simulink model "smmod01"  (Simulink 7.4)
settings: Solver=ode45  StartTime=0.0  StopTime=3  MaxStep=5e-4  RelTol=1e-4  AbsTol=1e-4
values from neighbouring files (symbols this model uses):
  Bm = 0.10    (= 0.1)    [IMabc2.m]    (also in imabcparam.m = 0.01; IMabcrun0.m = 0.01; IMabcrun1.m = 0.001; IMcur0.m = 1e-06)
  H = 0.60    (= 0.6)    [IMabc2.m]    (also in IMcur0.m = 0.3; imdef0vec.m = 0.3; imdef1vec.m = 0.3; imdef2vec.m = 0.3)
  n0 = 0.98    [imdef0vec.m]    (also in imdef1vec.m = 0.978; imdef2vec.m; imdefrotflux.m; imdefSIvec1.m = 0.95)
  Ra = .95    (= 0.95)    [altwdgs.m]    (also in Ccurverun.m = 0.018)
  Te0 = 0.75/wo*p*(Is*conj(Is)*Req)    [imdefSIvec1.m]
  V = [Vas 0 0].'    [Actac.m]    (also in acttrcalc1.m = str2num(get(h,'string')); im3d.m = eval(get(hVs,'String')); IMabc2.m = [vas vbs vcs 0 0 0]'; IMabcf0.m = [vas vbs vcs 0 0 0]')
  wo = 2*pi*freq0    [calc0.m]    (also in IMabc2.m = 376.991118431; imabcparam.m = 376.991118431; IMabcrun0.m = 376.991118431; IMabcrun1.m = 376.991118431)
undefined symbols (not defined in the file or in its folder): delta0, fa0, fk0, Lal, Lfl, Lkdl, Lkql, Lmd, Lmq, ph, phif0, Rf, Rkd, Rkq, vf0

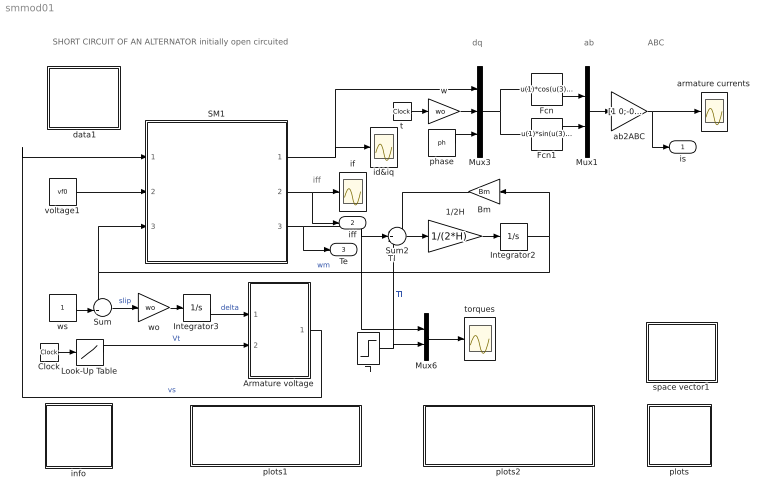
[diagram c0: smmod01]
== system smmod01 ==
  note: Tl
  note: SHORT CIRCUIT OF AN ALTERNATOR initially open circuited
  note: iff
  note: dq
  note: ab
  note: ABC
  " data1" : Subsystem
  1/2H : Gain  Gain=1/(2*H)  ParameterDataType=sfix(16)  ParameterScaling=2^0  OutDataType=sfix(16)  OutScaling=2^0
  Armature voltage : Subsystem
  Bm : Gain  Gain=Bm  ParameterDataType=sfix(16)  ParameterScaling=2^0  OutDataType=sfix(16)  OutScaling=2^0
  Clock : Clock
  Fcn : Fcn  Expr=u(1)*cos(u(3)+u(4))-u(2)*sin(u(3)+u(4))
  Fcn1 : Fcn  Expr=u(1)*sin(u(3)+u(4))+u(2)*cos(u(3)+u(4))
  Integrator2 : Integrator  InitialCondition=n0
  Integrator3 : Integrator  InitialCondition=delta0
  Look-Up Table : Lookup  InputValues=[0 0.2 0.2 5]  Table=[V V 0 0]  OutDataType=sfix(16)  OutScaling=2^0
  Mux1 : Mux  Inputs=2
  Mux3 : Mux  Inputs=3
  Mux6 : Mux  Inputs=2
  SM1 : Subsystem
  Sum : Sum  Inputs=-+|  OutDataType=sfix(16)  OutScaling=2^0
  Sum2 : Sum  Inputs=-+-  OutDataType=sfix(16)  OutScaling=2^0
  Tl : Step  Time=0  After=Te0  SampleTime=0
  ab2ABC : Gain  Gain=[1 0;-0.5 sqrt(3)/2;-0.5 -sqrt(3)/2]  Multiplication=Matrix(K*u)  ParameterDataType=sfix(16)  ParameterScaling=2^0  OutDataType=sfix(16)  OutScaling=2^0
  armature currents : Scope
  id&iq : Scope
  if : Scope
  info : Subsystem
  phase : Constant  Value=ph  OutDataType=sfix(16)  OutScaling=2^0
  plots : Subsystem
  plots1 : Subsystem
  plots2 : Subsystem
  space vector1 : Subsystem
  t : Clock
  torques : Scope
  voltage1 : Constant  Value=vf0  OutDataType=sfix(16)  OutScaling=2^0
  w : Gain  Gain=wo  ParameterDataType=sfix(16)  ParameterScaling=2^0  OutDataType=sfix(16)  OutScaling=2^0
  wo : Gain  Gain=wo  ParameterDataType=sfix(16)  ParameterScaling=2^0  OutDataType=sfix(16)  OutScaling=2^0
  ws : Constant  OutDataType=sfix(16)  OutScaling=2^0
  is : Outport
  iff : Outport  Port=2
  Te : Outport  Port=3
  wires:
  voltage1/1 -> SM1/2(vf)
  1/2H/1 -> Integrator2/1
  Sum2/1 -> 1/2H/1
  Bm/1 -> Sum2/1
  Mux6/1 -> torques/1
  ws/1 -> Sum/2
  Sum/1 -> wo/1  "slip"
  Armature voltage/1(vs) -> SM1/1(vs)  "vs"
  wo/1 -> Integrator3/1
  Integrator3/1 -> Armature voltage/1(delta)  "delta"
  Clock/1 -> Look-Up Table/1
  Look-Up Table/1 -> Armature voltage/2(Vt)  "Vt"
  Integrator2/1 -> Bm/1, Sum/1, SM1/3(wm)  "wm"
  w/1 -> Mux3/2
  phase/1 -> Mux3/3
  t/1 -> w/1
  SM1/2(if) -> if/1, iff/1
  SM1/3(Te) -> Sum2/2, Mux6/1, Te/1
  SM1/1(ia) -> id&iq/1, Mux3/1
  Tl/1 -> Mux6/2, Sum2/3  "Tl"
  Mux3/1 -> Fcn/1, Fcn1/1
  Fcn1/1 -> Mux1/2
  Fcn/1 -> Mux1/1
  Mux1/1 -> ab2ABC/1
  ab2ABC/1 -> armature currents/1, is/1

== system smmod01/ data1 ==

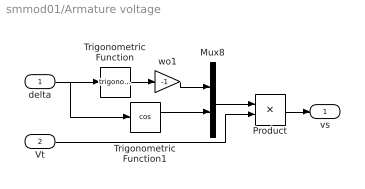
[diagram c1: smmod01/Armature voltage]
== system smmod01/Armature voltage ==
  delta : Inport  OutDataType=sfix(16)  OutScaling=2^0
  Vt : Inport  Port=2  OutDataType=sfix(16)  OutScaling=2^0
  Mux8 : Mux  Inputs=2
  Product : Product  OutDataType=sfix(16)  OutScaling=2^0
  Trigonometric Function : Trigonometry
  Trigonometric Function1 : Trigonometry  Operator=cos
  wo1 : Gain  Gain=-1  ParameterDataType=sfix(16)  ParameterScaling=2^0  OutDataType=sfix(16)  OutScaling=2^0
  vs : Outport
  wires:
  delta/1 -> Trigonometric Function/1, Trigonometric Function1/1
  Trigonometric Function/1 -> wo1/1
  Mux8/1 -> Product/1
  wo1/1 -> Mux8/1
  Trigonometric Function1/1 -> Mux8/2
  Product/1 -> vs/1
  Vt/1 -> Product/2

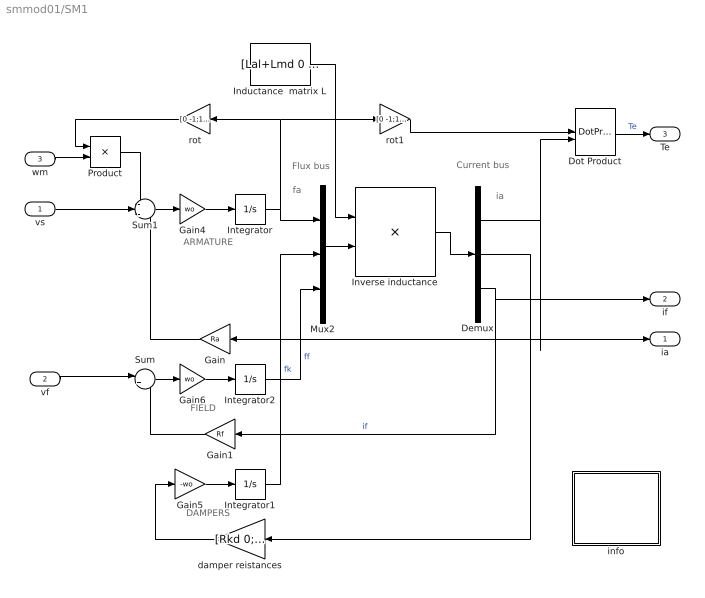
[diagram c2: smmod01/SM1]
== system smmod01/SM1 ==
  note: DAMPERS
  note: ARMATURE
  note: fa
  note: ia
  note: FIELD
  note: Flux bus
  note: Current bus
  vs : Inport  OutDataType=sfix(16)  OutScaling=2^0
  vf : Inport  Port=2  OutDataType=sfix(16)  OutScaling=2^0
  wm : Inport  Port=3  OutDataType=sfix(16)  OutScaling=2^0
  Demux : Demux  Outputs=3
  Dot Product : DotProduct  OutDataType=fixdt(1, 16)  OutScaling=2^-10
  Gain : Gain  Gain=Ra  ParameterDataType=sfix(16)  ParameterScaling=2^0  OutDataType=sfix(16)  OutScaling=2^0
  Gain1 : Gain  Gain=Rf  ParameterDataType=sfix(16)  ParameterScaling=2^0  OutDataType=sfix(16)  OutScaling=2^0
  Gain4 : Gain  Gain=wo  ParameterDataType=sfix(16)  ParameterScaling=2^0  OutDataType=sfix(16)  OutScaling=2^0
  Gain5 : Gain  Gain=-wo  ParameterDataType=sfix(16)  ParameterScaling=2^0  OutDataType=sfix(16)  OutScaling=2^0
  Gain6 : Gain  Gain=wo  ParameterDataType=sfix(16)  ParameterScaling=2^0  OutDataType=sfix(16)  OutScaling=2^0
  Inductance  matrix L : Constant  Value=[Lal+Lmd 0 Lmd 0 Lmd;0 Lal+Lmq 0 Lmq 0;Lmd 0 Lmd+Lkdl 0 Lmd;0 Lmq 0 Lmq+Lkql 0;Lmd 0 Lmd 0 Lmd+Lfl]  VectorParams1D=off  OutDataType=fixdt(1, 16)  OutScaling=2^0
  Integrator : Integrator  InitialCondition=fa0
  Integrator1 : Integrator  InitialCondition=fk0
  Integrator2 : Integrator  InitialCondition=phif0
  Inverse inductance : Product  Inputs=/*  Multiplication=Matrix(*)  OutDataType=sfix(16)  OutScaling=2^0
  Mux2 : Mux  Inputs=3
  Product : Product  OutDataType=sfix(16)  OutScaling=2^0
  Sum : Sum  Inputs=|+-  OutDataType=sfix(16)  OutScaling=2^0
  Sum1 : Sum  Inputs=-+-  OutDataType=sfix(16)  OutScaling=2^0
  damper reistances : Gain  Gain=[Rkd 0;0 Rkq]  Multiplication=Matrix(K*u)  ParameterDataType=sfix(16)  ParameterScaling=2^0  OutDataType=sfix(16)  OutScaling=2^0
  info : Subsystem
  rot : Gain  Gain=[0 -1;1 0]  Multiplication=Matrix(K*u)  ParameterDataType=sfix(16)  ParameterScaling=2^0  OutDataType=sfix(16)  OutScaling=2^0
  rot1 : Gain  Gain=[0 -1;1 0]  Multiplication=Matrix(K*u)  ParameterDataType=sfix(16)  ParameterScaling=2^0  OutDataType=sfix(16)  OutScaling=2^0
  ia : Outport
  if : Outport  Port=2
  Te : Outport  Port=3
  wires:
  Product/1 -> Sum1/1
  rot/1 -> Product/1
  wm/1 -> Product/2
  Gain5/1 -> Integrator1/1
  damper reistances/1 -> Gain5/1
  Integrator/1 -> Mux2/1, rot/1, rot1/1
  Sum1/1 -> Gain4/1
  Gain4/1 -> Integrator/1
  vs/1 -> Sum1/2
  Gain/1 -> Sum1/3
  Gain6/1 -> Integrator2/1
  Sum/1 -> Gain6/1
  vf/1 -> Sum/1
  Gain1/1 -> Sum/2
  rot1/1 -> Dot Product/1
  Demux/1 -> Gain/1, ia/1, Dot Product/2
  Dot Product/1 -> Te/1  "Te"
  Integrator1/1 -> Mux2/2  "fk"
  Integrator2/1 -> Mux2/3  "ff"
  Demux/2 -> damper reistances/1
  Demux/3 -> if/1, Gain1/1  "if"
  Mux2/1 -> Inverse inductance/2
  Inductance  matrix L/1 -> Inverse inductance/1
  Inverse inductance/1 -> Demux/1

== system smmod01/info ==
  note: This demonstration illustrates the dynamics of a synchronous generator, initially open circuited, following a three-phase short circuit at the terminals. The electric dynamic model of the synchronous machine is represented by a fifth- order dynamic system accounting for the field and damper circuits as well as armature transients.
  note: Synchronous machine transients under shortcircuit

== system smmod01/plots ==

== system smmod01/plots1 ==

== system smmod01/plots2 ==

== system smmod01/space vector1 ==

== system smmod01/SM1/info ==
  note: This demonstration illustrates the dynamics of a synchronous generator, initially at no load, following a three-phase short circuit at the terminals.
  note: Synchronous machine transients under shortcircuit
